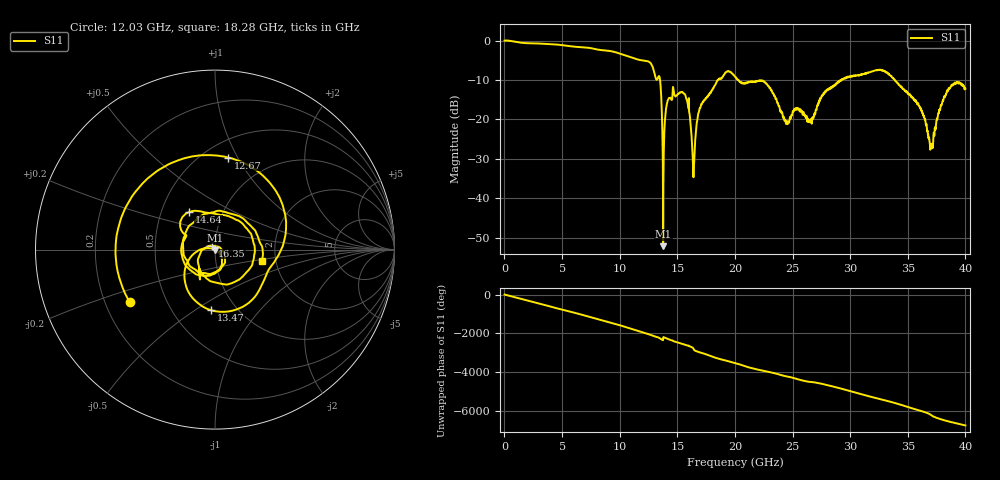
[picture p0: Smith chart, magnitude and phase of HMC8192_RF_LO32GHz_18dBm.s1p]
! Analog Devices, Inc.
! 1 Analog Way
! Wilmington, MA 01887
! http://www.analog.com
! Date:  2021-09-17 NN
! Board Name:  EVALHMC8192LG Revision A with HMC8192LG installed
! File Description:  S-Parameters for evaluation board without connectors or board loss de-embedded
! File Generation:  Calibrated Network Analyzer
! Chip Part Number:  HMC8192
! Chip Description:  Wideband IQ Mixer
! Chip Frequency:  20 to 42 GHz
! Chip Package:  LGA_CAV, 4 x 4 x 1.55 mm
! Chip State:
!  Temperature:  25C
!  LO Frequency:  32GHz
!  LO Power:  18dBm
! Note:
!  Analog Devices supplies this data as a sample of measured data at the evaluation board
!  ports for this product.  Your particular data for this product may vary.
!  Analog Devices reserves the right to change this data at anytime.
!  All lines below in this file are as is from the Network Analyzer.
!Keysight Technologies,N5245A,MY49151104,A.10.65.16
!Date: Tuesday, September 14, 2021 12:21:24
!Correction: S11(Full 2 Port(1,2))
!S1P File: Measurement: S11:
# Hz S  dB  R 50
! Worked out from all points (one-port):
!   3940 points, 10 MHz to 40 GHz, reference 50 ohm
!   lowest |S11| = -52.1 dB at 13.77 GHz (marker M1), VSWR 1.00, Z = 49.9 - j0.243 ohm
!   |S11| at or under -10 dB: 13.5 GHz to 18.54 GHz (5.037 GHz wide, 31.4 % of centre); 20.31 GHz to 29.23 GHz (8.915 GHz wide, 36 % of centre); 33.87 GHz to end of sweep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
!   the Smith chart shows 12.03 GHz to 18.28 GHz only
!   S11 on the Smith chart (normalised r, x): 12.03 GHz: 0.30, -0.26; 12.67 GHz: 0.65, +0.92; 13.47 GHz: 0.76, -0.58; 14.64 GHz: 0.69, +0.31; 16.35 GHz: 0.96, +0.04; 18.28 GHz: 1.70, -0.23
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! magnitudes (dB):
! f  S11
! 10 MHz  0.0
! 5.01 GHz  -1.2
! 10.01 GHz  -3.3
! 12.03 GHz  -5.1
! 12.67 GHz  -5.7
! 13.47 GHz  -9.4
! 13.77 GHz  -52.1
! 13.91 GHz  -20.8
! 14.14 GHz  -15.5
! 14.64 GHz  -11.9
! 15.01 GHz  -13.7
! 15.82 GHz  -15.0
! 16.35 GHz  -30.8
! 16.97 GHz  -17.1
! 18.28 GHz  -11.3
! 20.01 GHz  -9.2
! 22.51 GHz  -10.3
! 24.44 GHz  -21.1
! 25.01 GHz  -18.1
! 26.6 GHz  -20.1
! 27.83 GHz  -13.1
! 30.01 GHz  -9.1
! 32.79 GHz  -7.5
! 35.01 GHz  -13.4
! 36.23 GHz  -18.1
! 37.02 GHz  -26.2
! 38.46 GHz  -12.9
! 40 GHz  -12.2
